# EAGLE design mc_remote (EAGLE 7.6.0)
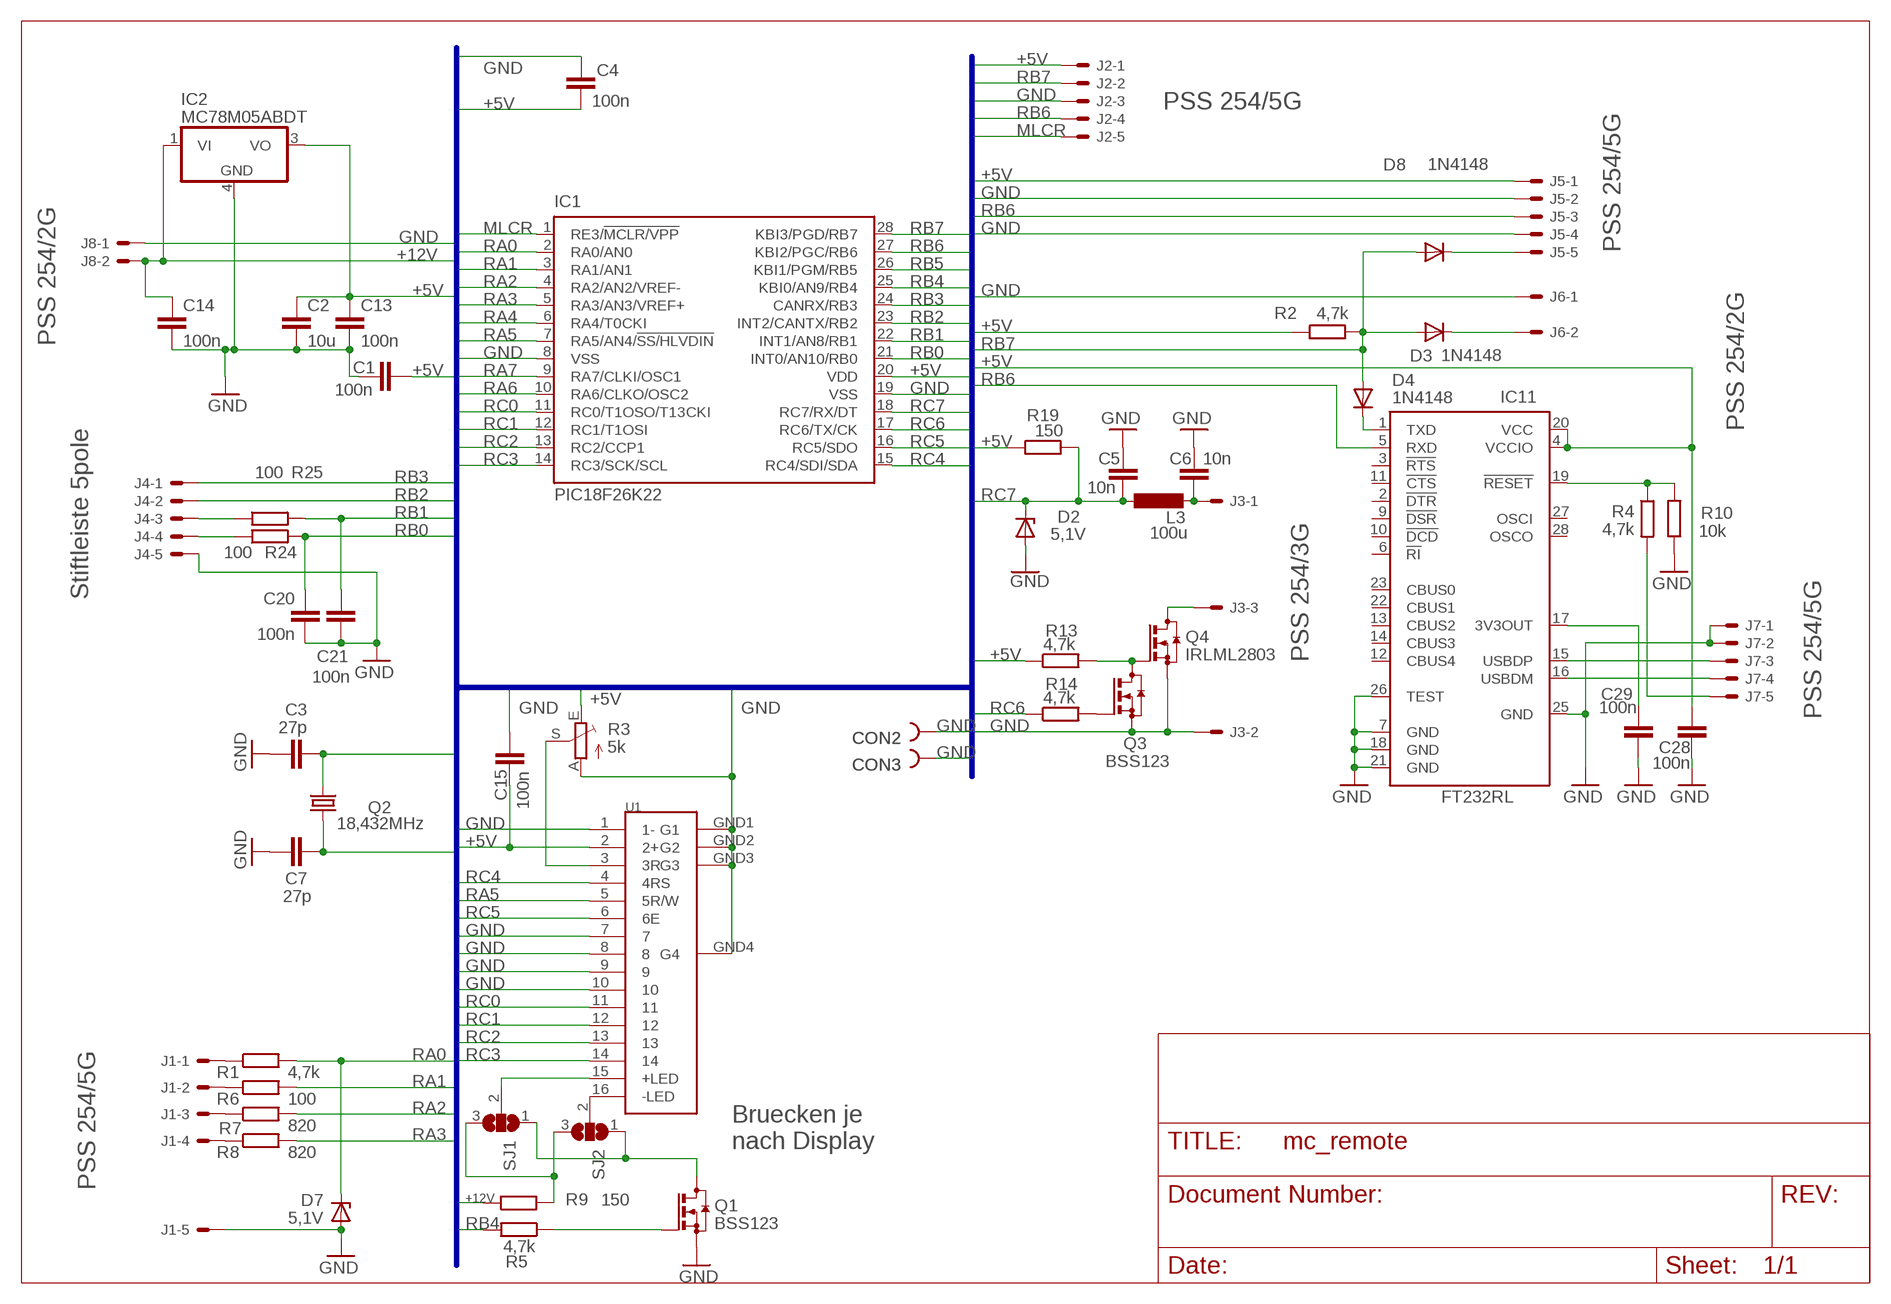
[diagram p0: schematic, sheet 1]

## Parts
C1  100n  C-EUC0805  [C0805]
C2  10u  C-EUC1206  [C1206]
C3  27p  C-EUC0805  [C0805]
C4  100n  C-EUC0805  [C0805]
C5  10n  C-EUC0805  [C0805]
C6  10n  C-EUC0805  [C0805]
C7  27p  C-EUC0805  [C0805]
C13  100n  C-EUC0805  [C0805]
C14  100n  C-EUC0805  [C0805]
C15  100n  C-EUC0805  [C0805]
C20  100n  C-EUC0805  [C0805]
C21  100n  C-EUC0805  [C0805]
C28  100n  C-EUC0805  [C0805]
C29  100n  C-EUC0805  [C0805]
CON2  PIN2_53MM  [HOLE3]
CON3  PIN2_53MM  [HOLE3]
D2  5,1V  ZENER-DIODESOT23  [SOT23]
D3  1N4148  DIODE-SOD323-W  [SOD323-W]
D4  1N4148  DIODE-SOD323-W  [SOD323-W]
D7  5,1V  ZENER-DIODESOT23  [SOT23]
D8  1N4148  DIODE-SOD323-W  [SOD323-W]
IC1  PIC18F26K22  PIC18F2480-I/SP  [DIL28-3]
IC2  MC78M05ABDT  [DPACK_3]
IC11  FT232RL  [SSOP28]
J1  PSS 254/5G  22-27-2051-05  [6410-05]
J2  PSS 254/5G  22-27-2051-05  [6410-05]
J3  PSS 254/3G  22-27-2031-03  [6410-03]
J4  Stiftleiste 5pole  22-27-2051-05  [6410-05]
J5  PSS 254/5G  22-27-2051-05  [6410-05]
J6  PSS 254/2G  22-27-2021-02  [6410-02]
J7  PSS 254/5G  22-27-2051-05  [6410-05]
J8  PSS 254/2G  22-27-2021-02  [6410-02]
L3  100u  L-EUL2825P  [L2825P]
Q1  BSS123  [SOT23]
Q2  18,432MHz  CRYSTALHC49S  [HC49/S]
Q3  BSS123  [SOT23]
Q4  IRLML2803  BSS123  [SOT23]
R1  4,7k  R-EU_M0805  [M0805]
R2  4,7k  R-EU_R0805  [R0805]
R3  5k  TRIM_EU-CA6V  [CA6V]
R4  4,7k  R-EU_M0805  [M0805]
R5  4,7k  R-EU_M0805  [M0805]
R6  100  R-EU_M0805  [M0805]
R7  820  R-EU_M0805  [M0805]
R8  820  R-EU_M0805  [M0805]
R9  150  R-EU_0309/10  [0309/10]
R10  10k  R-EU_R0805  [R0805]
R13  4,7k  R-EU_M0805  [M0805]
R14  4,7k  R-EU_M0805  [M0805]
R19  150  R-EU_M0805  [M0805]
R24  100  R-EU_M0805  [M0805]
R25  100  R-EU_M0805  [M0805]
SJ1  SJ2W  [SJ_2]
SJ2  SJ2W  [SJ_2]
U1  LCD_DOTNUR_OBEN  [LCD4X20_OBEN]

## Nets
+5V: C1.1 C2.1 C4.2 C13.1 C15.2 C28.1 IC1.20(VDD) IC2.3(VO) IC11.4(VCCIO) IC11.20(VCC) J2.1 J5.1 R2.1 R3.E R13.1 R19.1 U1.2(2+)
+12V: C14.1 IC2.1(VI) J8.2 R9.1
GND: C1.2 C2.2 C3.1 C4.1 C5.1 C6.1 C7.1 C13.2 C14.2 C15.1 C20.2 C21.2 C28.2 C29.2 CON2.1 CON3.1 D2.1(A) D7.1(A) IC1.8(VSS) IC1.19(VSS) IC2.4(GND) IC11.7(GND) IC11.18(GND) IC11.21(GND) IC11.25(GND) IC11.26(TEST) J1.5 J2.3 J3.2 J4.5 J5.2 J5.4 J6.1 J7.1 J7.2 J8.1 Q1.2(S) Q3.2(S) Q4.2(S) R3.A R10.1 U1.1(1-) U1.7 U1.8 U1.9 U1.10 U1.GND1(G1) U1.GND2(G2) U1.GND3(G3) U1.GND4(G4)
MLCR: IC1.1(RE3/!MCLR/VPP) J2.5
N$1: D8.C J5.5
N$2: J3.3 Q4.3(D)
N$3: D3.C J6.2
N$4: R3.S U1.3(3R)
N$5: D4.C IC11.1(TXD)
N$6: IC11.19(!RESET) R4.1 R10.2
N$7: Q1.1(G) R5.1
N$8: SJ2.2 U1.16(-LED)
N$9: SJ1.2 U1.15(+LED)
N$10: Q3.1(G) R14.2
N$11: J7.5 R4.2
N$12: J1.2 R6.1
N$13: J1.1 R1.1
N$14: C6.2 J3.1 L3.2
N$15: J1.3 R7.1
N$16: R9.2 SJ1.3 SJ2.3
N$17: Q1.3(D) SJ1.1 SJ2.1
N$18: Q3.3(D) Q4.1(G) R13.2
N$19: J1.4 R8.1
N$38: J4.4 R24.1
N$39: J4.3 R25.1
N$67: C29.1 IC11.17(3V3OUT)
N$68: IC11.15(USBDP) J7.3
N$69: IC11.16(USBDM) J7.4
RA0: D7.3(C) IC1.2(RA0/AN0) R1.2
RA1: IC1.3(RA1/AN1) R6.2
RA2: IC1.4(RA2/AN2/VREF-) R7.2
RA3: IC1.5(RA3/AN3/VREF+) R8.2
RA4: IC1.6(RA4/T0CKI)
RA5: IC1.7(RA5/AN4/!SS/HLVDIN) U1.5(5R/W)
RA6: C3.2 IC1.10(RA6/CLKO/OSC2) Q2.2
RA7: C7.2 IC1.9(RA7/CLKI/OSC1) Q2.1
RB0: C20.1 IC1.21(INT0/AN10/RB0) R24.2
RB1: C21.1 IC1.22(INT1/AN8/RB1) R25.2
RB2: IC1.23(INT2/CANTX/RB2) J4.2
RB3: IC1.24(CANRX/RB3) J4.1
RB4: IC1.25(KBI0/AN9/RB4) R5.2
RB5: IC1.26(KBI1/PGM/RB5)
RB6: IC1.27(KBI2/PGC/RB6) IC11.5(RXD) J2.4 J5.3
RB7: D3.A D4.A D8.A IC1.28(KBI3/PGD/RB7) J2.2 R2.2
RC0: IC1.11(RC0/T1OSO/T13CKI) U1.11
RC1: IC1.12(RC1/T1OSI) U1.12
RC2: IC1.13(RC2/CCP1) U1.13
RC3: IC1.14(RC3/SCK/SCL) U1.14
RC4: IC1.15(RC4/SDI/SDA) U1.4(4RS)
RC5: IC1.16(RC5/SDO) U1.6(6E)
RC6: IC1.17(RC6/TX/CK) R14.1
RC7: C5.2 D2.3(C) IC1.18(RC7/RX/DT) L3.1 R19.2
Unconnected: IC11.2(!DTR) IC11.3(!RTS) IC11.6(!RI) IC11.9(!DSR) IC11.10(!DCD) IC11.11(!CTS) IC11.12(CBUS4) IC11.13(CBUS2) IC11.14(CBUS3) IC11.22(CBUS1) IC11.23(CBUS0) IC11.27(OSCI) IC11.28(OSCO)

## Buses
+12V,+5V,GND,RA[0..7],RB[0..7],RC[0..7],RD[0..7],RE[0..2],MLCR

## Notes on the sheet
- Bruecken je 
  nach Display

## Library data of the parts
C1-C7 C13-C15 C20 C21 C28 C29 = rcl:C-EU: CAPACITOR, European symbol
CON2 CON3 = lindenau:PIN2_5
D2 D7 = diode:ZENER-DIODE: Z-Diode
D3 D4 D8 = diode:DIODE-: DIODE
IC1 = microchip:PIC18F2*80: 28-Pin Enhanced Flash Microcontrollers with ECAN(TM) Technology 10-Bit A/D and nanoWatt Technology Source: http://www.microchip.com .. 39637a.pdf; MF: MICROCHIP; MPN: PIC18F2480-I/SP; OC_FARNELL: 9321217; OC_NEWARK: 71J7237
IC2 = linear:MC78M: 500 mA Positive Voltage Regulators Source: Data sheet
IC11 = ftdichip:FT232R: Source: http://www.ftdichip.com/Documents/DataSheets/DS_FT232R_v104.pdf
J1 J2 J4 J5 J7 = con-molex:22-?-05: CONNECTOR wire to board 2.54 mm (.1 inch) pitch header; OC_FARNELL: unknown; OC_NEWARK: unknown
J3 = con-molex:22-?-03: CONNECTOR wire to board 2.54 mm (.1 inch) pitch header; OC_FARNELL: unknown; OC_NEWARK: unknown
J6 J8 = con-molex:22-?-02: CONNECTOR; OC_FARNELL: unknown; OC_NEWARK: unknown
L3 = rcl:L-EU: INDUCTOR, European symbol
Q1 Q3 Q4 = transistor-small-signal:BSS123: N-CHANNEL MOS FET
Q2 = crystal:CRYSTAL: CRYSTAL; OC_FARNELL: 1667008; OC_NEWARK: unknown
R1 R2 R4-R10 R13 R14 R19 R24 R25 = rcl:R-EU_: RESISTOR, European symbol
R3 = pot:TRIM_EU-: POTENTIOMETER
SJ1 SJ2 = jumper:SJ2W: SMD solder JUMPER
U1 = lindenau:LCD_DOT

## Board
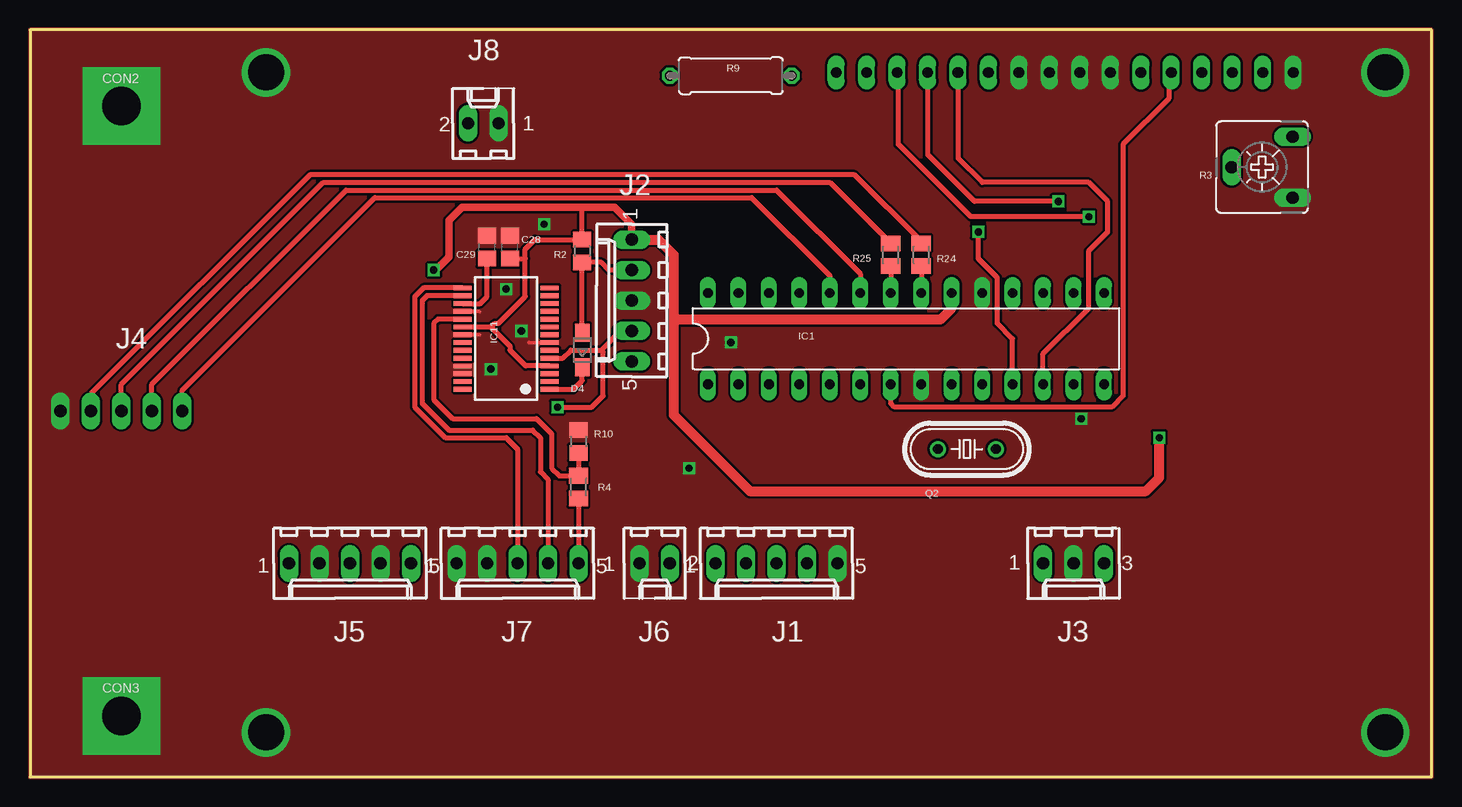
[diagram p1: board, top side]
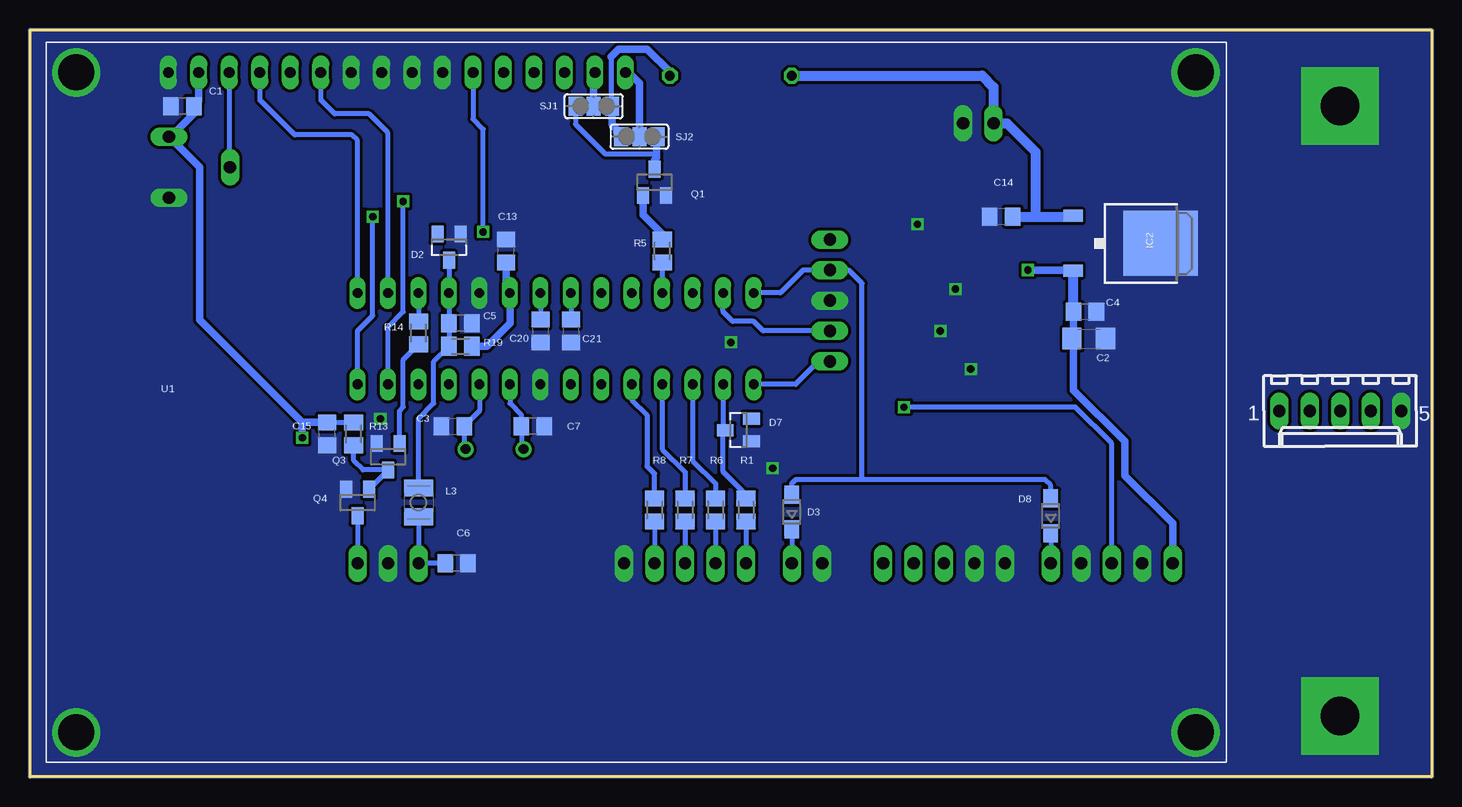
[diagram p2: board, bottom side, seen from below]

Size 116.84 x 62.23 mm. Coordinates in mm from the lower left corner, seen from the top.
Outline: 0,0 116.84,0 116.84,62.23 0,62.23 0,0
Copper layers (1*16): Top 0.035mm / dielectric 1.5mm / Bottom 0.035mm
Design rules "default *": minimum track width 10mil, minimum drill 24mil, track to track 8mil, track to pad 8mil, pad to pad 8mil, via to via 8mil, smd to smd 8mil, copper to edge 0mil, drill to drill 8mil, minimum pad ring 10mil, minimum via ring 8mil, stop-mask expansion 4mil, vias tented up to drill 0mil, thermal gap 10mil

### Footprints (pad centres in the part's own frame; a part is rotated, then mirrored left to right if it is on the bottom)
C0805 = smd 1.3 x 1.5: 1 -0.95,0; 2 0.95,0
C1206 = smd 1.6 x 1.8: 1 -1.4,0; 2 1.4,0
HOLE3 = drill 3.2 pad 6.452 square: 1 0,0
SOT23 = smd 1 x 1.4: 1 -0.95,-1.1; 2 0.95,-1.1; 3 0,1.1
SOD323-W = smd 1.5 x 1.2: A 1.45,0; C -1.45,0
DIL28-3 = drill 0.813 long: 1 -16.51,-3.81; 2 -13.97,-3.81; 3 -11.43,-3.81; 4 -8.89,-3.81; 5 -6.35,-3.81; 6 -3.81,-3.81; 7 -1.27,-3.81; 8 1.27,-3.81; 9 3.81,-3.81; 10 6.35,-3.81; 11 8.89,-3.81; 12 11.43,-3.81; 13 13.97,-3.81; 14 16.51,-3.81; 15 16.51,3.81; 16 13.97,3.81; 17 11.43,3.81; 18 8.89,3.81; 19 6.35,3.81; 20 3.81,3.81; 21 1.27,3.81; 22 -1.27,3.81; 23 -3.81,3.81; 24 -6.35,3.81; 25 -8.89,3.81; 26 -11.43,3.81; 27 -13.97,3.81; 28 -16.51,3.81
DPACK_3 = smd 1 x 1.6: 1 -2.28,-4.8; 3 2.28,-4.8 | smd 5.4 x 6.2: 4 0,2.5
SSOP28 = smd 0.4 x 1.5: 1 -4.225,-3.625; 2 -3.575,-3.625; 3 -2.925,-3.625; 4 -2.275,-3.625; 5 -1.625,-3.625; 6 -0.975,-3.625; 7 -0.325,-3.625; 8 0.325,-3.625; 9 0.975,-3.625; 10 1.625,-3.625; 11 2.275,-3.625; 12 2.925,-3.625; 13 3.575,-3.625; 14 4.225,-3.625; 15 4.225,3.625; 16 3.575,3.625; 17 2.925,3.625; 18 2.275,3.625; 19 1.625,3.625; 20 0.975,3.625; 21 0.325,3.625; 22 -0.325,3.625; 23 -0.975,3.625; 24 -1.625,3.625; 25 -2.275,3.625; 26 -2.925,3.625; 27 -3.575,3.625; 28 -4.225,3.625
6410-05 = drill 1.016 long: 1 5.08,0; 2 2.54,0; 3 0,0; 4 -2.54,0; 5 -5.08,0
6410-03 = drill 1.016 long: 1 2.54,0; 2 0,0; 3 -2.54,0
6410-02 = drill 1.016 long: 1 1.27,0; 2 -1.27,0
L2825P = smd 1.4 x 2.4: 1 -1.2,0; 2 1.2,0
HC49/S = drill 0.813: 1 -2.413,0; 2 2.413,0
M0805 = smd 1.3 x 1.6: 1 -0.95,0; 2 0.95,0
R0805 = smd 1.3 x 1.5: 1 -0.95,0; 2 0.95,0
CA6V = drill 1.016 long: A -2.54,-2.54; E 2.54,-2.54; S 0,2.54
0309/10 = drill 0.813 octagon: 1 -5.08,0; 2 5.08,0
SJ_2 = smd 1.168 x 1.6: 1 -1.524,0; 2 0,0; 3 1.524,0
LCD4X20_OBEN = drill 0.9 long: 1 10.265,57.419; 2 12.805,57.419; 3 15.345,57.419; 4 17.885,57.419; 5 20.425,57.419; 6 22.965,57.419; 7 25.505,57.419; 8 28.045,57.419; 9 30.585,57.419; 10 33.125,57.419; 11 35.665,57.419; 12 38.205,57.419; 13 40.745,57.419; 14 43.285,57.419; 15 45.825,57.419; 16 48.365,57.419 | drill 3: GND1 2.582,57.419; GND2 95.9,57.419; GND3 95.9,2.419; GND4 2.582,2.419

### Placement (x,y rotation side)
C1  104.14,55.88 180 bottom
C2  28.57,36.51 0 bottom
C3  81.6,29.21 0 bottom
C4  28.89,38.73 180 bottom
C5  80.96,37.78 180 bottom
C6  81.28,17.78 180 bottom
C7  74.93,29.21 180 bottom
C13  77.15,43.81 90 bottom
C14  35.88,46.67 180 bottom
C15  92.08,28.57 90 bottom
C20  74.3,37.15 270 bottom
C21  71.75,37.15 270 bottom
C28  40.01,44.13 90 top
C29  38.1,44.13 90 top
CON2  7.62,55.88 0 top
CON3  7.62,5.08 0 top
D2  81.92,44.13 180 bottom
D3  53.34,22.07 90 bottom
D4  46.04,35.56 90 top
D7  57.78,28.89 90 bottom
D8  31.75,21.75 90 bottom
IC1  73.03,36.51 0 top
IC2  25.08,44.45 270 bottom
IC11  39.69,36.51 90 top
J1  62.23,17.78 180 top
J2  50.16,39.69 90 top
J3  87,17.78 180 top
J4  7.62,30.48 180 bottom
J5  26.67,17.78 180 top
J6  52.07,17.78 180 top
J7  40.64,17.78 180 top
J8  37.78,54.45 0 top
L3  84.45,22.86 270 bottom
Q1  64.77,49.53 0 bottom
Q2  78.11,27.3 0 top
Q3  87,26.67 180 bottom
Q4  89.53,22.86 180 bottom
R1  57.15,22.23 90 bottom
R2  46.04,43.81 270 top
R3  102.71,50.8 90 top
R4  45.72,24.13 270 top
R5  64.14,43.81 270 bottom
R6  59.69,22.23 90 bottom
R7  62.23,22.23 90 bottom
R8  64.77,22.23 90 bottom
R9  58.42,58.42 0 top
R10  45.72,27.94 270 top
R13  89.85,28.57 270 bottom
R14  84.45,36.99 270 bottom
R19  80.96,35.88 180 bottom
R24  74.3,43.5 270 top
R25  71.75,43.5 270 top
SJ1  69.85,55.88 0 bottom
SJ2  66.04,53.34 180 bottom
U1  115.57,1.27 0 bottom

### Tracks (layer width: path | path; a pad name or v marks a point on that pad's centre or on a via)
+5V  (via drill 0.6)
  Top 0.406: 38.4,37.49 IC11.20 38.44,37.49 38.73,37.78 39.05,37.78 41.27,40.01 41.27,43.18 | 38.4,37.49 40.01,35.88 40.01,35.56 41.33,34.24 IC11.4 | 38.42,37.51 38.4,37.49 | R2.1 | C28.1 41.27,43.18 | R2.1 46.04,47.31 45.88,47.47 | 41.27,43.18 41.27,43.97 42.07,44.77 R2.1
  Top 0.61: J2.1 50.16,46.04 48.74,47.47 45.88,47.47 36.04,47.47 34.92,46.35 34.92,43.34 33.81,42.23 v33.66,42.23
  Top 0.813: J2.1 52.39,44.77 53.66,43.5 53.66,38.1 | 53.66,38.1 53.66,30.16 60.01,23.81 93.03,23.81 94.14,24.92 v94.14,28.26 | 53.66,38.1 75.88,38.1 76.83,39.05 IC1.20
  Bottom 0.406: C15.2 R13.1 | C4.2 29.98,38.73 C2.1
  Bottom 0.61: C13.1 77.15,40.64 IC1.20 76.83,37.78 78.74,35.88 R19.1 79.22,35.88 | C15.2 94.14,29.53 | 94.14,29.53 102.71,38.1 102.71,50.8 R3.E 105.09,53.34 103.19,55.24 C1.1 102.77,56.3 U1.2 | v94.14,28.26 94.14,29.53 | C4.2 29.84,32.22 25.56,27.94 25.56,25.08 21.59,21.11 J5.1 | v33.66,42.23 29.94,42.23 IC2.3
  Bottom 0.813: C4.2 29.84,42.17 IC2.3
+12V
  Bottom 0.813: C14.1 33.02,46.67 | 33.02,46.67 29.88,46.67 IC2.1 | 33.02,46.67 33.02,52.07 35.4,54.45 J8.2 36.51,57.47 37.47,58.42 R9.1
GND  (via drill 0.6)
  Top 0.305: IC11.21 37.46,36.84 37.47,36.83 | IC11.18 37.41,38.79 37.47,38.73 | IC11.7 41.6,36.19 41.59,36.2
  other vias: 87.63,29.84 58.42,36.2 39.69,40.64 42.86,46.04 40.96,37.15 38.42,33.97 54.93,25.72
  pour Bottom (isolate 0.254, no thermals): 0,62.23 0,0 116.84,0 116.84,62.23
  pour Top (no thermals): 0,62.23 0,0 116.84,0 116.84,62.23
MLCR
  Bottom 0.406: J2.5 51.12,34.61 53.02,32.7 IC1.1
N$1
  Bottom 0.406: D8.C J5.5
N$2
  Bottom 0.406: Q4.3 J3.3
N$3
  Bottom 0.406: D3.C J6.2
N$4
  Bottom 0.406: U1.3 100.22,50.85 R3.S
N$5
  Top 0.406: IC11.1 45.3,32.29 46.04,33.02 D4.C
N$6
  Top 0.406: IC11.19 34.01,38.14 33.66,37.78 33.66,31.43 35.24,29.84 42.23,29.84 43.5,28.57 43.5,25.72 44.13,25.08 R4.1 R10.2
N$7
  Bottom 0.61: R5.1 64.14,45.24 65.72,46.83 Q1.1
N$8
  Bottom 0.61: U1.16 66.94,58.69 66.04,57.78 SJ2.2
N$9
  Bottom 0.61: U1.15 69.85,58.69 SJ1.2
N$10
  Bottom 0.406: Q3.1 86.05,30.48 85.72,30.8 85.72,34.77 R14.2
N$11
  Top 0.406: R4.2 J7.5
N$12
  Bottom 0.406: R6.1 J1.2
N$13
  Bottom 0.406: R1.1 J1.1
N$14
  Bottom 0.406: L3.2 J3.1 C6.2
N$15
  Bottom 0.406: R7.1 J1.3
N$16
  Bottom 0.406: 68.42,60.01 68.42,55.98 SJ1.3
  Bottom 0.61: SJ1.3 68.33,54.36 67.94,53.98 67.94,53.72 SJ2.3 | R9.2 63.5,58.74 65.41,60.64 67.79,60.64 68.42,60.01
N$17
  Bottom 0.406: SJ1.1 71.37,54.39 68.9,51.91 64.61,51.91
  Bottom 0.61: Q1.3 64.77,51.44 64.61,51.59 64.61,51.91 64.61,53.24 SJ2.1
N$18
  Bottom 0.406: Q4.1 87,25.55 Q3.3 89.07,25.57 89.85,26.35 R13.2
N$19
  Bottom 0.406: R8.1 J1.4
N$38
  Top 0.406: J4.4 5.08,31.91 23.34,50.16 68.74,50.16 74.3,44.61 R24.1
N$39
  Top 0.406: J4.3 7.62,32.7 24.45,49.53 66.67,49.53 R25.1
N$67
  Top 0.406: IC11.17 37.53,39.44 38.1,40.01 C29.1
N$68
  Top 0.406: IC11.15 32.8,40.74 32.07,40.01 32.07,30.8 34.61,28.26 39.69,28.26 40.64,27.3 J7.3
N$69
  Top 0.406: IC11.16 33.1,40.09 32.7,39.69 32.7,31.11 34.92,28.89 41.91,28.89 42.55,28.26 42.55,25.4 43.18,24.77 J7.4
RA0
  Bottom 0.406: R1.2 57.15,23.5 59.05,25.4 59.05,28.72 D7.3 59.05,29.06 IC1.2
RA1
  Bottom 0.406: IC1.3 61.59,26.35 59.69,24.45 R6.2
RA2
  Bottom 0.406: IC1.4 64.14,27.3 62.23,25.4 R7.2
RA3
  Bottom 0.406: IC1.5 66.67,31.43 65.41,30.16 65.41,25.89 64.77,25.25 R8.2
RA5
  Top 0.406: U1.5 94.93,58.48 94.93,56.52 91.12,52.7 91.12,31.75 90.17,30.8 72.07,30.8 71.75,31.11 IC1.7
RA6
  Bottom 0.406: IC1.10 79.38,30.48 C3.2 80.65,27.43 Q2.2
RA7
  Bottom 0.406: IC1.9 76.83,31.11 75.88,30.16 C7.2 75.88,27.49 Q2.1
RB0
  Top 0.406: R24.2 IC1.21
  Bottom 0.406: IC1.21 C20.1
RB1
  Top 0.406: R25.2 IC1.22
  Bottom 0.406: IC1.22 C21.1
RB2
  Top 0.406: J4.2 10.16,32.7 26.35,48.9 62.23,48.9 69.22,41.91 IC1.23
RB3
  Top 0.406: J4.1 12.7,32.23 28.73,48.26 60.17,48.26 66.67,41.75 IC1.24
RB4
  Bottom 0.406: R5.2 IC1.25
RB6  (via drill 0.6)
  Top 0.406: IC11.5 44.41,34.89 45.09,35.56 47.62,35.56 | 47.62,35.56 49.21,37.15 J2.4 | v43.97,30.8 46.83,30.8 47.78,31.75 47.78,35.4 47.62,35.56
  Bottom 0.406: J5.3 26.67,27.78 29.69,30.8 v43.97,30.8 | J2.4 55.72,37.15 56.52,37.94 58.26,37.94 59.05,38.73 IC1.27
RB7
  Top 0.406: D4.A R2.2 47.62,42.86 48.26,42.23 J2.2
  Bottom 0.406: D8.A 31.75,24.29 32.23,24.77 47.62,24.77 | 47.62,24.77 53.02,24.77 53.34,24.45 D3.A | 47.62,24.77 47.47,24.92 47.47,41.12 48.58,42.23 J2.2 52.39,42.23 54.29,40.32 IC1.28
RC0  (via drill 0.6)
  Top 0.406: IC1.11 81.92,36.51 80.64,37.78 80.64,41.59 79.06,43.18 v79.06,45.4
  Bottom 0.406: v79.06,45.4 79.06,53.98 79.91,54.82 U1.11
RC1
  Top 0.406: IC1.12 84.45,35.24 88.27,39.05 88.27,43.81 89.85,45.4 89.85,47.94 88.27,49.53 79.38,49.53 77.36,51.54 U1.12
RC2  (via drill 0.6)
  Top 0.406: v85.72,47.94 78.74,47.94 74.83,51.86 U1.13
  Bottom 0.406: IC1.13 87,37.47 85.72,38.73 v85.72,47.94
RC3  (via drill 0.6)
  Top 0.406: v88.27,46.67 78.42,46.67 72.39,52.7 72.39,58.58 U1.14
  Bottom 0.406: IC1.14 89.53,37.15 88.27,38.42 v88.27,46.67
RC4
  Bottom 0.406: U1.4 97.69,56.41 94.77,53.5 90.01,53.5 89.53,53.02 IC1.15
RC5
  Bottom 0.406: IC1.16 87,53.66 88.58,55.24 91.44,55.24 92.61,56.41 U1.6
RC6
  Bottom 0.406: IC1.17 R14.1
RC7
  Bottom 0.406: D2.3 IC1.18 C5.2 R19.2 83.19,34.6 83.19,31.11 84.45,29.84 L3.1

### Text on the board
Document: SV 12V | Programmer | Dreh_Taste | RS232 | USB extern | RS232 zum PicAStar | LEDadc | RS232 PicATU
